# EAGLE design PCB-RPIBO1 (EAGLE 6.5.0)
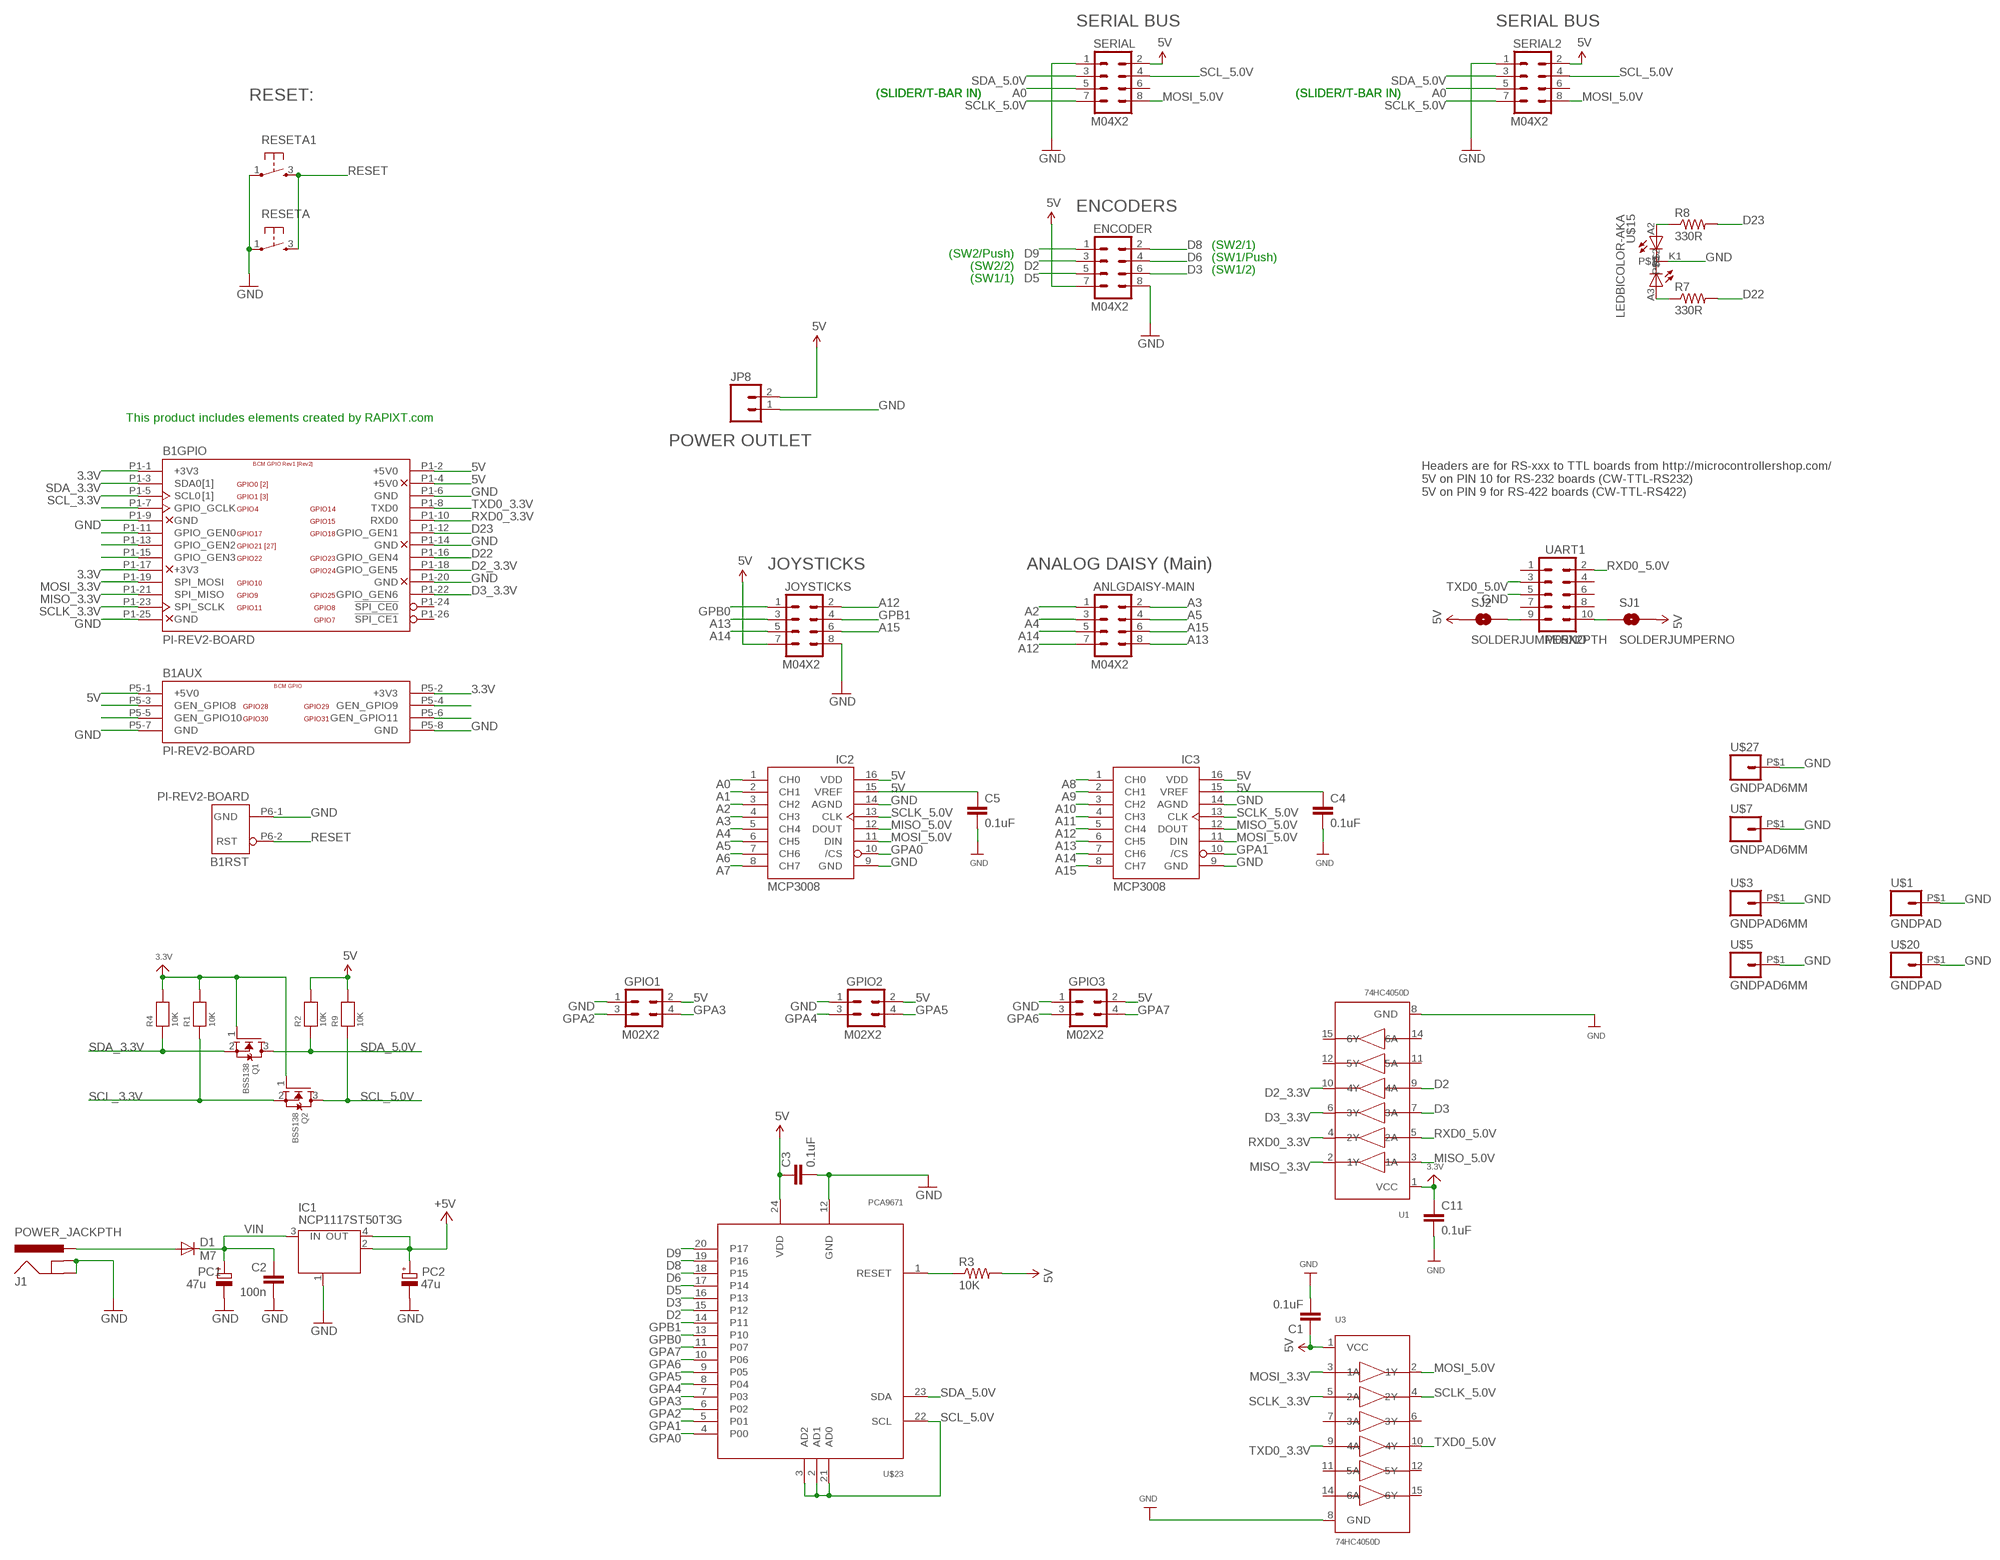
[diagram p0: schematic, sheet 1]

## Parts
ANLGDAISY-MAIN  M04X2  [2X4]
B1  PI-REV2-BOARD  [RASPBERRY-PI-REV2]
C1  0.1uF  CAP0603-CAP  [0603-CAP]
C2  100n  C-EU0603-RND  [C0603-ROUND]
C3  0.1uF  CAP0603-CAP  [0603-CAP]
C4  0.1uF  CAP0603-CAP  [0603-CAP]
C5  0.1uF  CAP0603-CAP  [0603-CAP]
C11  0.1uF  CAP0603-CAP  [0603-CAP]
D1  M7  DIODE-SMB  [SMB]
ENCODER  M04X2  [2X4]
GPIO1  M02X2  [2X2]
GPIO2  M02X2  [2X2]
GPIO3  M02X2  [2X2]
IC1  NCP1117ST50T3G  MC33269ST-3.3T3  [SOT223]
IC2  MCP3008  [DIL16]
IC3  MCP3008  [DIL16]
J1  POWER_JACKPTH  [POWER_JACK_PTH]
JOYSTICKS  M04X2  [2X4]
JP8  M02PTH4  [1X02_XTRA_BIG]
PC1  47u  CPOL-EUD  [PANASONIC_D]
PC2  47u  CPOL-EUD  [PANASONIC_D]
Q1  BSS138  MOSFET-NWIDE  [SOT23-WIDE]
Q2  BSS138  MOSFET-NWIDE  [SOT23-WIDE]
R1  10K  RESISTOR0805  [0805]
R2  10K  RESISTOR0805  [0805]
R3  10K  RESISTOR0603-RES  [0603-RES]
R4  10K  RESISTOR0805  [0805]
R7  330R  RESISTOR0603-RES  [0603-RES]
R8  330R  RESISTOR0603-RES  [0603-RES]
R9  10K  RESISTOR0805  [0805]
RESETA  TAC_SWITCH  [PUSHBUTTON]
RESETA1  TAC_SWITCH  [PUSHBUTTON]
SERIAL  M04X2  [2X4]
SERIAL2  M04X2  [2X4]
SJ1  SOLDERJUMPERNO  [SJ_2S-NO]
SJ2  SOLDERJUMPERNO  [SJ_2S-NO]
U1  74HC4050D  [SOIC16]
U3  74HC4050D  [SOIC16]
U$1  GNDPAD  [3.2MMPAD]
U$3  GNDPAD6MM  [3.2MMPAD6MM]
U$5  GNDPAD6MM  [3.2MMPAD6MM]
U$7  GNDPAD6MM  [3.2MMPAD6MM]
U$15  LEDBICOLOR-AKA  [LED5MM-BICOLOR]
U$20  GNDPAD  [3.2MMPAD]
U$23  PCA9671  [TSSOP24]
U$27  GNDPAD6MM  [3.2MMPAD6MM]
UART1  M05X2PTH  [AVR_ICSP]

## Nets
3.3V [Power]: B1.P1-1(GPIO:+3V3) B1.P1-17(GPIO:+3V3) B1.P5-2(AUX:+3V3) C11.1 Q1.1(G) Q2.1(G) R1.2 R4.2 U1.1(VCC)
5V [Power]: B1.P1-2(GPIO:+5V0) B1.P1-4(GPIO:+5V0) B1.P5-1(AUX:+5V0) C1.1 C3.1 C4.1 C5.1 ENCODER.7 GPIO1.2 GPIO2.2 GPIO3.2 IC1.2(OUT) IC1.4(OUT) IC2.15(VREF) IC2.16(VDD) IC3.15(VREF) IC3.16(VDD) JOYSTICKS.7 JP8.2 PC2.+ R2.2 R3.2 R9.2 SERIAL2.2 SERIAL.2 SJ1.2 SJ2.1 U3.1(VCC) U$23.24(VDD) ; supply symbol labelled +5V
12V [Power]: D1.A J1.PWR
A0: IC2.1(CH0) SERIAL2.5 SERIAL.5
A1: IC2.2(CH1)
A2: ANLGDAISY-MAIN.1 IC2.3(CH2)
A3: ANLGDAISY-MAIN.2 IC2.4(CH3)
A4: ANLGDAISY-MAIN.3 IC2.5(CH4)
A5: ANLGDAISY-MAIN.4 IC2.6(CH5)
A6: IC2.7(CH6)
A7: IC2.8(CH7)
A8: IC3.1(CH0)
A9: IC3.2(CH1)
A10: IC3.3(CH2)
A11: IC3.4(CH3)
A12: ANLGDAISY-MAIN.7 IC3.5(CH4) JOYSTICKS.2
A13: ANLGDAISY-MAIN.8 IC3.6(CH5) JOYSTICKS.3
A14: ANLGDAISY-MAIN.5 IC3.7(CH6) JOYSTICKS.5
A15: ANLGDAISY-MAIN.6 IC3.8(CH7) JOYSTICKS.6
D2: ENCODER.3 U1.9(4A) U$23.15(P12)
D2_3.3V: B1.P1-18(GPIO:GPIO_GEN5) U1.10(4Y)
D3: ENCODER.6 U1.7(3A) U$23.16(P13)
D3_3.3V: B1.P1-22(GPIO:GPIO_GEN6) U1.6(3Y)
D5: ENCODER.5 U$23.17(P14)
D6: ENCODER.4 U$23.18(P15)
D8: ENCODER.2 U$23.19(P16)
D9: ENCODER.1 U$23.20(P17)
D22: B1.P1-16(GPIO:GPIO_GEN4) R7.2
D23: B1.P1-12(GPIO:GPIO_GEN1) R8.2
GND [Power]: B1.P1-6(GPIO:GND) B1.P1-9(GPIO:GND) B1.P1-14(GPIO:GND) B1.P1-20(GPIO:GND) B1.P1-25(GPIO:GND) B1.P5-7(AUX:GND) B1.P5-8(AUX:GND) B1.P6-1(RST:GND) C1.2 C2.2 C3.2 C4.2 C5.2 C11.2 ENCODER.8 GPIO1.1 GPIO2.1 GPIO3.1 IC1.1(GND/ADJ) IC2.9(GND) IC2.14(AGND) IC3.9(GND) IC3.14(AGND) J1.GND J1.SHUNT(GNDBREAK) JOYSTICKS.8 JP8.1 PC1.- PC2.- RESETA1.1 RESETA.1 SERIAL2.1 SERIAL.1 U1.8(GND) U3.8(GND) U$1.P$1 U$3.P$1 U$5.P$1 U$7.P$1 U$15.K1 U$20.P$1 U$23.12(GND) U$27.P$1 UART1.5
GPA0: IC2.10(/CS) U$23.4(P00)
GPA1: IC3.10(/CS) U$23.5(P01)
GPA2: GPIO1.3 U$23.6(P02)
GPA3: GPIO1.4 U$23.7(P03)
GPA4: GPIO2.3 U$23.8(P04)
GPA5: GPIO2.4 U$23.9(P05)
GPA6: GPIO3.3 U$23.10(P06)
GPA7: GPIO3.4 U$23.11(P07)
GPB0: JOYSTICKS.1 U$23.13(P10)
GPB1: JOYSTICKS.4 U$23.14(P11)
MISO_3.3V: B1.P1-21(GPIO:SPI_MISO) U1.2(1Y)
MISO_5.0V: IC2.12(DOUT) IC3.12(DOUT) U1.3(1A)
MOSI_3.3V: B1.P1-19(GPIO:SPI_MOSI) U3.3(1A)
MOSI_5.0V: IC2.11(DIN) IC3.11(DIN) SERIAL2.8 SERIAL.8 U3.2(1Y)
N$1: R3.1 U$23.1(RESET)
N$9: SJ2.2 UART1.9
N$10: SJ1.1 UART1.10
N$17: R8.1 U$15.A2
N$22: R7.1 U$15.A3
N$23: B1.P1-15(GPIO:GPIO_GEN3)
N$24: B1.P1-13(GPIO:GPIO_GEN2)
N$25: B1.P1-11(GPIO:GPIO_GEN0)
N$27: B1.P1-7(GPIO:GPIO_GCLK)
N$34: B1.P5-4(AUX:GEN_GPIO9)
N$35: B1.P5-6(AUX:GEN_GPIO11)
N$38: B1.P5-3(AUX:GEN_GPIO8)
N$39: B1.P5-5(AUX:GEN_GPIO10)
RESET: B1.P6-2(RST:RST) RESETA1.3 RESETA.3
RXD0_3.3V: B1.P1-10(GPIO:RXD0) U1.4(2Y)
RXD0_5.0V: U1.5(2A) UART1.2
SCL_3.3V: B1.P1-5(GPIO:SCL0) Q2.2(S) R1.1
SCL_5.0V: Q2.3(D) R9.1 SERIAL2.4 SERIAL.4 U$23.2(AD1) U$23.3(AD2) U$23.21(AD0) U$23.22(SCL)
SCLK_3.3V: B1.P1-23(GPIO:SPI_SCLK) U3.5(2A)
SCLK_5.0V: IC2.13(CLK) IC3.13(CLK) SERIAL2.7 SERIAL.7 U3.4(2Y)
SDA_3.3V: B1.P1-3(GPIO:SDA0) Q1.2(S) R4.1
SDA_5.0V: Q1.3(D) R2.1 SERIAL2.3 SERIAL.3 U$23.23(SDA)
TXD0_3.3V: B1.P1-8(GPIO:TXD0) U3.9(4A)
TXD0_5.0V: U3.10(4Y) UART1.3
VIN [Power]: C2.1 D1.C IC1.3(IN) PC1.+
Unconnected: B1.P1-24(GPIO:!SPI_CE0) B1.P1-26(GPIO:!SPI_CE1) SERIAL2.6 SERIAL.6 U1.11(5A) U1.12(5Y) U1.14(6A) U1.15(6Y) U3.6(3Y) U3.7(3A) U3.11(5A) U3.12(5Y) U3.14(6A) U3.15(6Y) UART1.1 UART1.4 UART1.6 UART1.7 UART1.8

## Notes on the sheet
- SERIAL BUS | SERIAL BUS
- (SLIDER/T-BAR IN) | (SLIDER/T-BAR IN) | (SLIDER/T-BAR IN) | (SLIDER/T-BAR IN)
- RESET:
- ENCODERS
- (SW2/Push) | (SW2/1)
- (SW2/2) | (SW1/Push)
- (SW1/1) | (SW1/2)
- This product includes elements created by RAPIXT.com
- POWER OUTLET
- Headers are for RS-xxx to TTL boards from http://microcontrollershop.com/
  5V on PIN 10 for RS-232 boards (CW-TTL-RS232)
  5V on PIN 9 for RS-422 boards (CW-TTL-RS422)
- JOYSTICKS | ANALOG DAISY (Main)

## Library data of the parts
ANLGDAISY-MAIN ENCODER JOYSTICKS SERIAL SERIAL2 = SparkFun:M04X2
B1 = SKAARHOJ:PI-REV2-: Raspberry Pi Rev2
C1 C3-C5 C11 = SparkFun:CAP: Capacitor
C2 = SmartPrj:C-EU: CAPACITOR, European symbol
D1 = diode:DIODE-: DIODE
GPIO1-GPIO3 = SKAARHOJ:M02X2
IC1 = linear:MC33269ST*: Adjustable Output Low Dropout Voltage Regulator 800 mA Source: http://www.onsemi.com/pub/Collateral/MC33269-D.PDF
IC2 IC3 = adafruit:MCP3008
J1 = SKAARHOJ:POWER_JACK: RASM712PX Right Angle SMT Mount DC Power Jack, pin size 0.100"(2.5mm), with locating post Switchcraft.com
JP8 = SparkFun:M02: Header 2
PC1 PC2 = rcl:CPOL-EU: POLARIZED CAPACITOR, European symbol
Q1 Q2 = microbuilder:MOSFET-N: N-Channel Mosfet LEGEND VDS: Voltage Drain-Source ID: Drain Current RDS(ON): Drain-Source On-State Resistance VGS(TH): Gate-Source Threshold Voltage CISS: Drain-Source Input Capacitance SOT-23 Name VDS ID RDS(ON) VGS(TH) CISS Order Number 2N7002E 60V 260mA 2.5 Ohm 2.5V @ 250uA 26.7pF @ 25V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
R1 R2 R4 R9 = microbuilder:RESISTOR: Resistors
R3 R7 R8 = SparkFun:RESISTOR: Resistor
RESETA RESETA1 = SKAARHOJ:TAC_SWITCH: Momentary Switch
SJ1 SJ2 = SparkFun:SOLDERJUMPER: Solder Jumper
U1 U3 = microbuilder:74HC4050D: 6-channel level shifter 74HC4050D - 2V-6V Supply Digikey: 74HC4050D,653-ND Mouser: 771-74HC4050D-T
U$1 U$3 U$5 U$7 U$20 U$27 = SKAARHOJ:GNDPAD
U$15 = SKAARHOJ:LEDBICOLOR-AKA
U$23 = SKAARHOJ:PCA9671
UART1 = SparkFun:M05X2: Header 5x2 Standard 10-pin dual row 0.1" header. Commonly used with AVR-ISP. Use with Spark Fun Electronics SKU: PRT-00778

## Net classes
0 default: width 0.203 mm, drill 0.406 mm, clearance 0.152 mm
1 Power: width 0.508 mm, drill 0.61 mm, clearance 0.203 mm
3 INput lines: clearance 0.203 mm

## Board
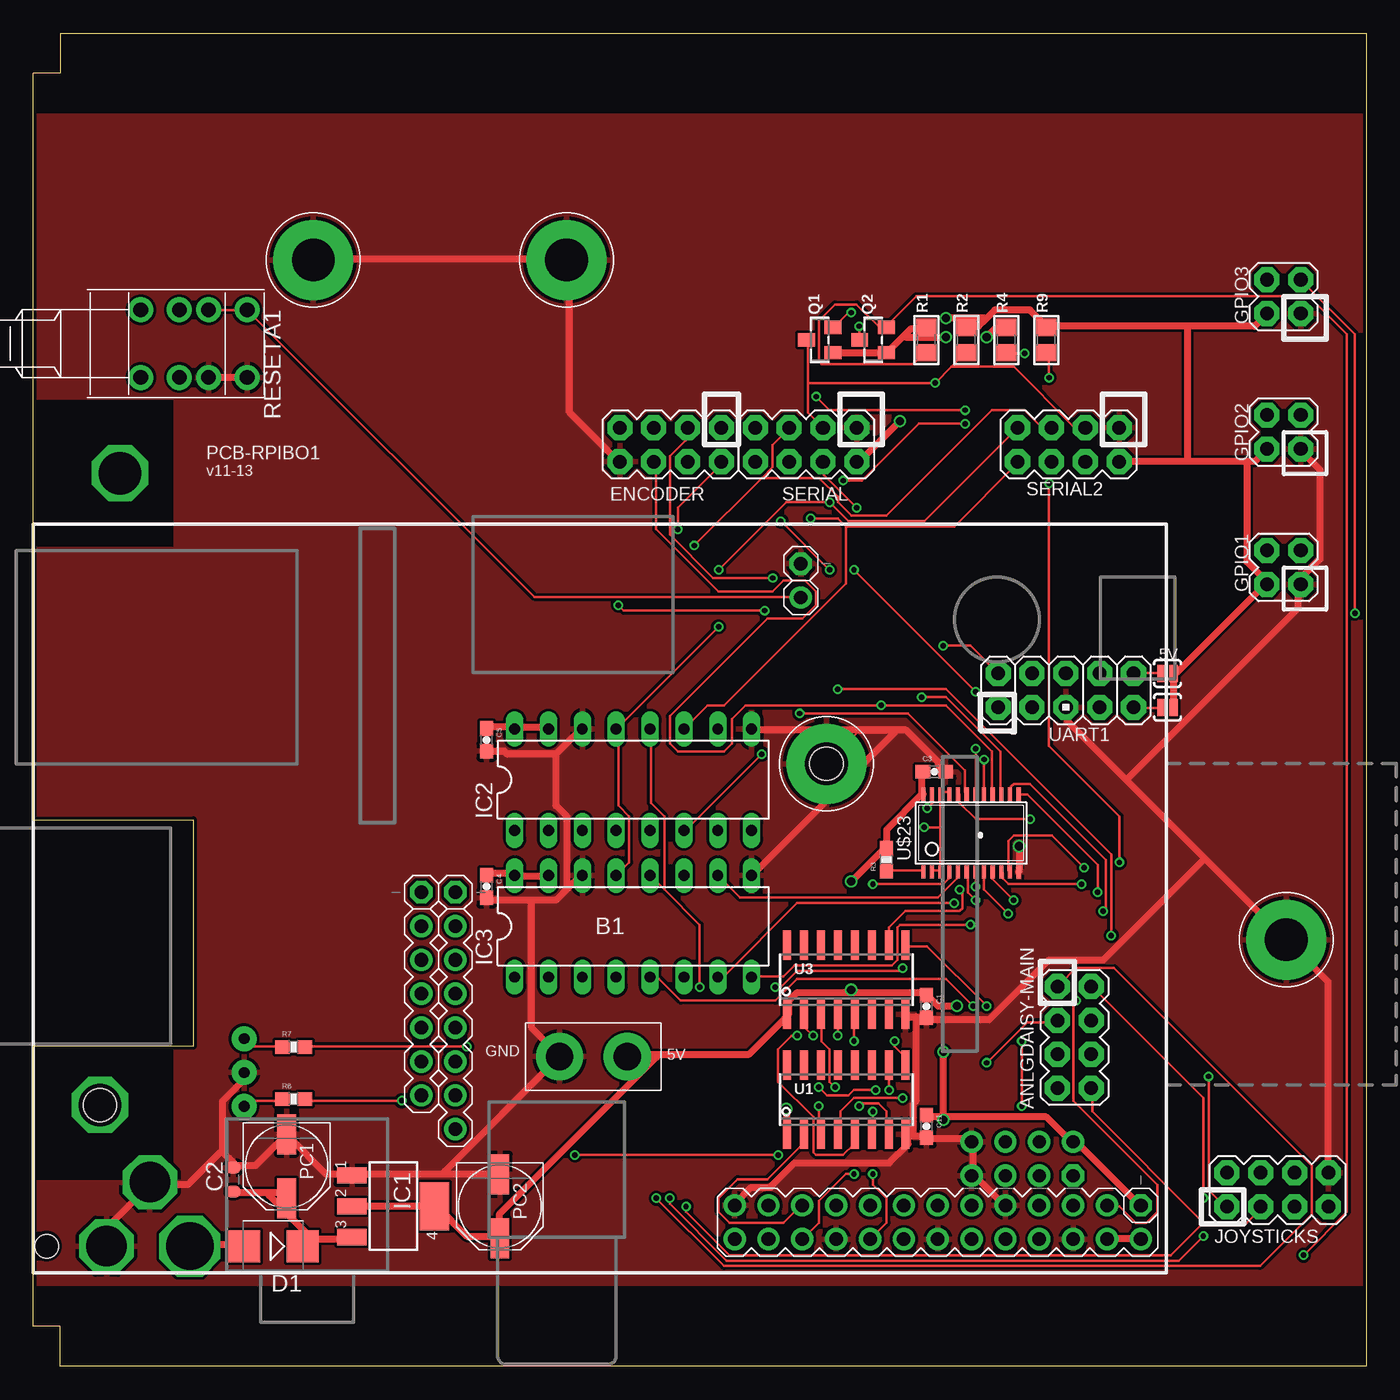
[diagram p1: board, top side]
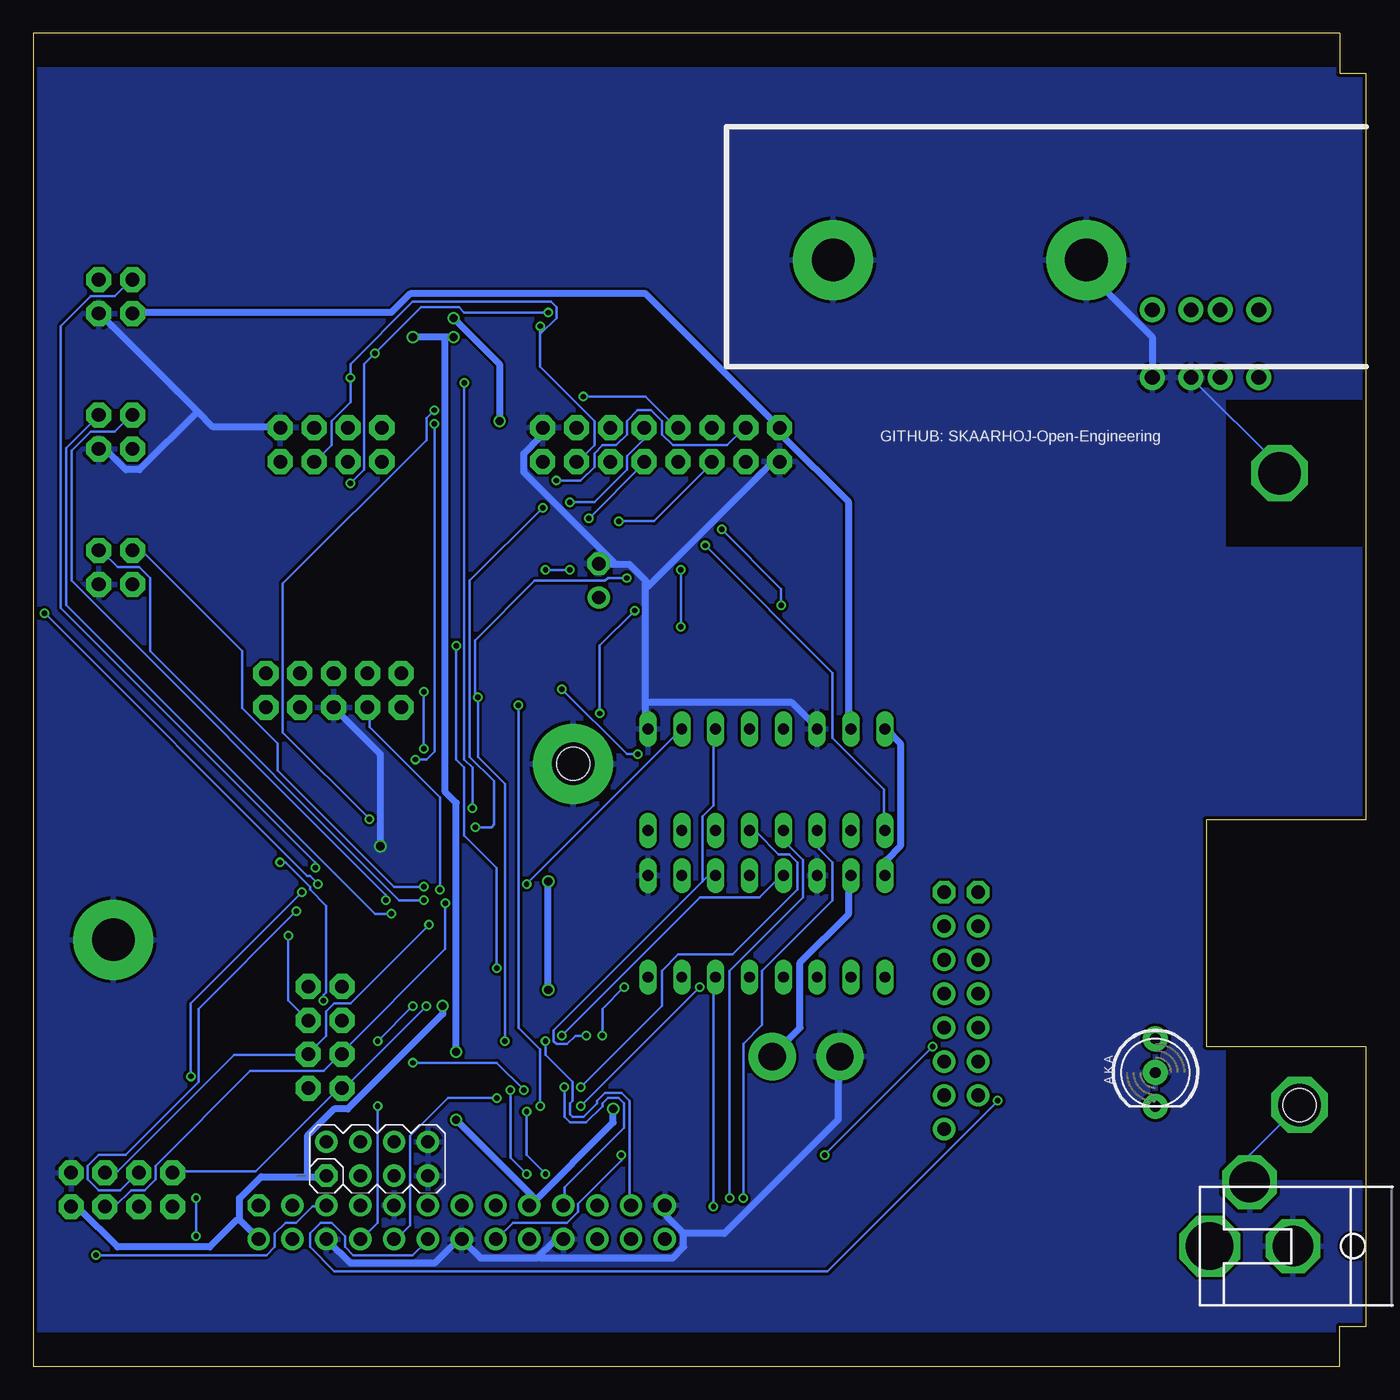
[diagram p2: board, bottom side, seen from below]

Size 100 x 100 mm. Coordinates in mm from the lower left corner, seen from the top.
Outline: 0,3 0,24 12,24 12,41 0,41 0,97 2,97 2,100 100,100 100,0 2,0 2,3 0,3
Copper layers (1*16): Top 0.035mm / dielectric 1.5mm / Bottom 0.035mm
Design rules "Fusion_eagle_rule_v1.1": minimum track width 6mil, minimum drill 12mil, track to track 6mil, track to pad 6mil, pad to pad 6mil, via to via 6mil, smd to smd 0mil, copper to edge 10mil, drill to drill 10mil, minimum pad ring 10mil, minimum via ring 6mil, stop-mask expansion 2mil, vias tented up to drill 100mil, thermal gap 10mil
tRestrict: area 0,14 to 10.5,25; area 0,61.5 to 10.5,72.5; area 0,94 to 100,100; area 0,0 to 100,6
bRestrict: area 0,61.5 to 10.5,72.5; area 0,14 to 10.5,25; area 0,0 to 100,2.5; area 0,97.5 to 100,100

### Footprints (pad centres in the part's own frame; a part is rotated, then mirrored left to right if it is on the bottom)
2X4 = drill 1.016 pad 1.88 octagon: 1 -3.81,-1.27; 2 -3.81,1.27; 3 -1.27,-1.27; 4 -1.27,1.27; 5 1.27,-1.27; 6 1.27,1.27; 7 3.81,-1.27; 8 3.81,1.27
RASPBERRY-PI-REV2 = drill 1.016 pad 1.676 octagon: P1-1 83.095,5.065; P2-1 31.66,28.56; P3-1 29.12,28.56 | drill 1.016 pad 1.676: P1-2 83.095,2.525; P1-3 80.555,5.065; P1-4 80.555,2.525; P1-5 78.015,5.065; P1-6 78.015,2.525; P1-7 75.475,5.065; P1-8 75.475,2.525; P1-9 72.935,5.065; P1-10 72.935,2.525; P1-11 70.395,5.065; P1-12 70.395,2.525; P1-13 67.855,5.065; P1-14 67.855,2.525; P1-15 65.315,5.065; P1-16 65.315,2.525; P1-17 62.775,5.065; P1-18 62.775,2.525; P1-19 60.235,5.065; P1-20 60.235,2.525; P1-21 57.695,5.065; P1-22 57.695,2.525; P1-23 55.155,5.065; P1-24 55.155,2.525; P1-25 52.615,5.065; P1-26 52.615,2.525; P2-2 31.66,26.02; P2-3 31.66,23.48; P2-4 31.66,20.94; P2-5 31.66,18.4; P2-6 31.66,15.86; P2-7 31.66,13.32; P2-8 31.66,10.78; P3-2 29.12,26.02; P3-3 29.12,23.48; P3-4 29.12,20.94; P3-5 29.12,18.4; P3-6 29.12,15.86; P3-7 29.12,13.32 | drill 1 pad 1.676 octagon: P5-1 78.015,7.287; P6-1 57.58,53.21 | drill 1 pad 1.676: P5-2 78.015,9.828; P5-3 75.475,7.287; P5-4 75.475,9.828; P5-5 72.935,7.287; P5-6 72.935,9.828; P5-7 70.395,7.287; P5-8 70.395,9.828; P6-2 57.58,50.67 | hole 2.5: 59.5,38.2; 5,12.6
0603-CAP = smd 1.1 x 1: 1 -0.85,0; 2 0.85,0
C0603-ROUND = smd 0.898 x 1.1: 1 -0.889,0; 2 0.889,0
SMB = smd 2.4 x 2.4: A 2.2,0; C -2.2,0
2X2 = drill 1.016 pad 1.88 octagon: 1 -3.81,-1.27; 2 -3.81,1.27; 3 -1.27,-1.27; 4 -1.27,1.27
SOT223 = smd 1.219 x 2.235: 1 -2.311,-3.099; 2 0,-3.099; 3 2.311,-3.099 | smd 3.6 x 2.2: 4 0,3.099
DIL16 = drill 0.813 long: 1 -8.89,-3.81; 2 -6.35,-3.81; 3 -3.81,-3.81; 4 -1.27,-3.81; 5 1.27,-3.81; 6 3.81,-3.81; 7 6.35,-3.81; 8 8.89,-3.81; 9 8.89,3.81; 10 6.35,3.81; 11 3.81,3.81; 12 1.27,3.81; 13 -1.27,3.81; 14 -3.81,3.81; 15 -6.35,3.81; 16 -8.89,3.81
POWER_JACK_PTH = drill 3.048 octagon: GND -7.493,0; SHUNT -10.744,4.801 | drill 3.556 octagon: PWR -13.741,0 | hole 1.778: -2.997,0
1X02_XTRA_BIG = drill 2.057 pad 3.556: 1 -2.54,0; 2 2.54,0
PANASONIC_D = smd 3 x 1.4: + 2.4,0; - -2.4,0
SOT23-WIDE = smd 1 x 1.27: 1 -0.95,-1; 2 0.95,-1; 3 0,1
0805 = smd 1.3 x 1.5: 1 -0.95,0; 2 0.95,0
0603-RES = smd 1.1 x 1: 1 -0.85,0; 2 0.85,0
PUSHBUTTON = drill 1.1 pad 1.88: 1 2.54,2.54; 2 2.54,-2.54; 3 -2.54,2.54; 4 -2.54,-2.54
SJ_2S-NO = smd 0.635 x 1.27: 1 -0.45,0; 2 0.45,0
SOIC16 = smd 0.6 x 2.2: 1 -4.445,-2.6; 2 -3.175,-2.6; 3 -1.905,-2.6; 4 -0.635,-2.6; 5 0.635,-2.6; 6 1.905,-2.6; 7 3.175,-2.6; 8 4.445,-2.6; 9 4.445,2.6; 10 3.175,2.6; 11 1.905,2.6; 12 0.635,2.6; 13 -0.635,2.6; 14 -1.905,2.6; 15 -3.175,2.6; 16 -4.445,2.6
3.2MMPAD = drill 3.2 octagon: P$1 0,0
3.2MMPAD6MM = drill 3.2 pad 6: P$1 0,0
LED5MM-BICOLOR = drill 0.813 pad 1.88: A2 2.54,0; A3 -2.54,0; K1 0,0
TSSOP24 = smd 0.305 x 0.991: 1 -4.225,-2.918; 2 -3.575,-2.918; 3 -2.925,-2.918; 4 -2.275,-2.918; 5 -1.625,-2.918; 6 -0.975,-2.918; 7 -0.325,-2.918; 8 0.325,-2.918; 9 0.975,-2.918; 10 1.625,-2.918; 11 2.275,-2.918; 12 2.925,-2.918; 13 2.925,2.918; 14 2.275,2.918; 15 1.625,2.918; 16 0.975,2.918; 17 0.325,2.918; 18 -0.325,2.918; 19 -0.975,2.918; 20 -1.625,2.918; 21 -2.275,2.918; 22 -2.925,2.918; 23 -3.575,2.918; 24 -4.225,2.918
AVR_ICSP = drill 1.016 pad 1.88 octagon: 1 -1.27,5.08; 2 1.27,5.08; 3 -1.27,2.54; 4 1.27,2.54; 5 -1.27,0; 6 1.27,0; 7 -1.27,-2.54; 8 1.27,-2.54; 9 -1.27,-5.08; 10 1.27,-5.08

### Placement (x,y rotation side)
ANLGDAISY-MAIN  78.11,24.67 270 top
B1  0,7 0 top
C1  67,27 270 top
C2  15,14 90 top
C3  67.6,44.6 0 top
C4  34,36 270 top
C5  34,47 270 top
C11  67,18 270 top
D1  18,9 180 top
ENCODER  47.81,69.14 180 top
GPIO1  93.83,62.47 90 top
GPIO2  93.83,72.63 90 top
GPIO3  93.83,82.79 90 top
IC1  27,12 270 top
IC2  45,44 0 top
IC3  45,33 0 top
J1  -2,9 0 bottom
JOYSTICKS  93.36,13.24 0 top
JP8  42.02,23.23 0 top
PC1  19,15 270 top
PC2  35,12 270 top
Q1  59,77 90 top
Q2  63,77 90 top
R1  67,77 90 top
R2  70,77 90 top
R3  64,38 90 top
R4  73,77 90 top
R7  19.52,23.95 0 top
R8  19.52,20.05 0 top
R9  76,77 90 top
RESETA  10.6,76.72 270 top
RESETA1  13.5,76.72 270 top
SERIAL  57.98,69.14 180 top
SERIAL2  77.66,69.14 180 top
SJ1  85.09,51.98 0 top
SJ2  85.09,49.44 180 top
U1  61,20 0 top
U3  61,29 0 top
U$1  6.5,67 0 top
U$3  21,83 0 top
U$5  40,83 0 top
U$7  94,32 0 top
U$15  15.81,22.03 270 bottom
U$20  5,19.6 0 top
U$23  71,40 0 top
U$27  59.5,45.2 0 top
UART1  77.47,50.7 90 top

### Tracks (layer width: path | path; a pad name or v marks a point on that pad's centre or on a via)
3.3V  (via drill 0.61)
  Top 0.508: v56.49,19.3 56.49,17.48 U1.1 | Q1.1 60.15,76 63.8,76 Q2.1 64.21,76.2 65.33,77.32 | 65.33,77.32 65.84,77.83 66.85,77.83 R1.2 | v71.53,77.22 72.14,77.83 72.95,77.83 R4.2 | v68.48,77.22 65.43,77.22 65.33,77.32 | 68.28,18.69 76,18.69 77.83,16.87 B1.P5-2 78.23,16.87 82.91,12.19 B1.P1-1 | 68.28,18.69 67.06,18.69 C11.1 | 68.28,18.69 v68.28,23.57 | v68.28,18.49 68.28,18.69
  Bottom 0.508: v56.49,19.3 56.49,18.29 62.59,12.19 B1.P1-17 62.38,12.6 v68.28,18.49 | v68.48,77.22 69.09,77.22 | 69.09,77.22 v71.53,77.22 | 69.09,77.22 69.09,43.08 68.28,42.27 v68.28,23.57
5V  (via drill 0.61)
  Top 0.508: SJ2.1 85.55,49.58 85.55,51.82 SJ1.2 85.75,52.02 92.46,58.73 GPIO1.2 92.46,58.93 91.03,60.35 91.03,67.87 | 91.03,67.87 91.64,67.87 92.46,68.68 GPIO2.2 | 91.03,67.87 86.56,67.87 | 86.56,67.87 81.48,67.87 SERIAL2.2 | 71.42,78.54 72.14,79.25 74.78,79.25 76,78.03 R9.2 76.2,78.03 86.56,78.03 | 71.42,78.54 70.92,78.03 70.1,78.03 R2.2 | 86.56,78.03 91.64,78.03 92.46,78.84 GPIO3.2 | v65.02,70.92 61.98,67.87 SERIAL.2 | v68.48,78.64 71.32,78.64 71.42,78.54 | 86.56,78.03 86.56,67.87 | C4.1 34.14,36.98 35.97,36.98 IC3.16 36.17,36.78 38.61,36.78 IC3.15 | C5.1 34.14,47.95 35.97,47.95 IC2.16 36.17,47.95 38.61,47.95 IC2.15 | B1.P1-4 80.67,9.55 82.91,9.55 B1.P1-2 | IC1.2 23.98,11.99 30.07,11.99 IC1.4 30.28,11.99 32.51,9.75 34.95,9.75 PC2.+ 34.95,9.96 34.95,11.38 46.74,23.16 46.74,23.37 | C3.1 66.65,44.5 66.65,43.08 U$23.24 66.65,42.88 64.01,40.23 64.01,39.01 R3.2 63.8,38.81 v61.37,36.37 | 61.37,28.04 57.3,28.04 56.69,27.43 56.69,26.42 U3.1 56.49,26.21 53.65,23.37 46.74,23.37 | 61.37,28.04 66.85,28.04 C1.1 67.06,27.84 67.87,27.03 v69.29,27.03 | v61.37,28.25 61.37,28.04 | 46.74,23.37 44.7,23.37 JP8.2
  Bottom 0.508: v65.02,70.92 65.02,75.18 v68.48,78.64 | IC2.15 38.81,47.95 38.81,64.82 43.89,69.9 43.89,70.31 ENCODER.7 44.09,70.51 54.05,80.47 71.73,80.47 73.15,79.05 92.46,79.05 GPIO3.2 | IC3.16 35.97,36.98 35.97,38 34.95,39.01 34.95,46.74 35.97,47.75 IC2.16 | 79.45,14.22 82.91,14.22 84.53,12.6 84.53,10.97 | 79.45,14.22 78.03,14.22 B1.P5-1 | 84.53,10.97 83.11,9.55 B1.P1-2 | JOYSTICKS.7 97.13,11.79 96.52,11.79 93.67,8.94 86.77,8.94 84.73,10.97 84.53,10.97 | v61.37,28.25 v61.37,36.37 | 79.45,14.22 79.45,17.27 77.42,19.3 76.4,19.3 69.29,26.42 v69.29,27.03 | IC3.15 38.81,36.78 38.81,33.93 42.47,30.28 42.47,25.4 44.5,23.37 JP8.2
12V
  Top 0.508: D1.A 15.65,9.14 11.79,9.14 J1.PWR
A0  (via drill 0.41)
  Top 0.203: 54.66,66.65 55.47,67.46 55.47,69.09 56.69,70.31 SERIAL.5 | 54.66,66.65 v49.58,61.57 | 54.66,66.65 58.93,66.65 60.35,65.23 60.35,64.82 61.37,63.8 64.01,63.8 71.93,71.73 74.37,71.73 75.59,70.51 76.2,70.51 SERIAL2.5
  Bottom 0.203: v49.58,61.57 40.03,52.02 40.03,47.14 36.17,43.28 36.17,40.23 IC2.1
A2  (via drill 0.41)
  Top 0.203: v46.74,12.6 51.82,7.52 92.05,7.52 95.91,11.38 95.91,15.04 81.08,29.87 78.23,29.87 77.01,28.65 ANLGDAISY-MAIN.1
  Bottom 0.203: v46.74,12.6 46.74,24.18 45.31,25.6 45.31,29.67 40.03,34.95 40.03,37.8 41.05,38.81 41.05,40.03 IC2.3
A3  (via drill 0.41)
  Top 0.203: v47.75,12.6 47.75,12.19 52.02,7.92 85.95,7.92 v87.78,9.75 | v87.78,12.6 87.78,20.12 79.45,28.45 ANLGDAISY-MAIN.2
  Bottom 0.203: v47.75,12.6 47.75,29.67 42.27,35.15 42.27,38 43.69,39.42 43.69,40.03 IC2.4 | v87.78,12.6 v87.78,9.75
A4  (via drill 0.41)
  Top 0.203: v58.93,20.93 59.54,20.32 61.16,20.32 61.57,20.73 v63.2,20.73 | v71.53,22.76 74.57,25.81 76.81,25.81 ANLGDAISY-MAIN.3
  Bottom 0.203: v58.93,20.93 52.83,27.03 52.83,29.67 51.61,30.89 47.55,30.89 42.67,35.76 42.67,37.8 43.28,38.41 44.09,38.41 45.72,40.03 46.13,40.03 IC2.5 | v63.2,20.73 65.23,22.76 v71.53,22.76
A5  (via drill 0.41)
  Top 0.203: v54.66,45.92 48.97,40.23 IC2.6 | v60.35,50.8 68.48,50.8 80.87,38.41 v80.87,32.31
  Bottom 0.203: v54.66,45.92 55.47,45.92 v60.35,50.8 | v80.87,32.31 80.87,27.43 79.45,26.01 ANLGDAISY-MAIN.4
A12  (via drill 0.41)
  Top 0.203: v70.51,27.03 68.48,29.06 57.3,29.06 55.68,27.43 48.56,27.43 46.94,29.06 46.33,29.06 IC3.5
  Bottom 0.203: v70.51,27.03 76.81,20.73 ANLGDAISY-MAIN.7 77.01,20.93 83.31,14.63 89.41,14.63 JOYSTICKS.2
A13  (via drill 0.41)
  Top 0.203: v48.97,11.99 48.97,11.58 52.22,8.33 85.34,8.33 87.78,10.77 | 87.78,10.77 91.03,10.77 92.05,11.79 JOYSTICKS.3 | 87.78,10.77 79.45,19.1 79.45,20.73 ANLGDAISY-MAIN.8
  Bottom 0.203: v48.97,11.99 48.97,29.06 IC3.6
A14  (via drill 0.41)
  Top 0.203: v69.09,34.75 57.3,34.75 51.82,29.26 51.41,29.26 IC3.7
  Bottom 0.203: v69.09,34.75 69.09,31.29 76.81,23.57 ANLGDAISY-MAIN.5 77.01,23.37 78.23,22.15 83.72,22.15 90.83,15.04 90.83,14.02 91.64,13.21 92.66,13.21 93.88,11.99 94.49,11.99 JOYSTICKS.5
A15  (via drill 0.41)
  Top 0.203: v70.31,33.12 65.02,33.12 64.82,32.92 64.82,30.48 64.41,30.07 57.1,30.07 56.29,29.26 54.05,29.26 IC3.8
  Bottom 0.203: v70.31,33.12 76.2,27.23 77.42,27.23 78.03,26.62 78.03,24.79 79.25,23.57 ANLGDAISY-MAIN.6 79.45,23.37 84.94,23.37 93.67,14.63 94.49,14.63 JOYSTICKS.6
D2  (via drill 0.41)
  Top 0.203: v66.65,50.19 68.48,50.19 72.54,46.13 72.54,43.08 U$23.15 | v64.62,24.38 64.62,23.98 65.43,23.16 65.43,22.76 U1.9 | v55.47,59.13 51,59.13 47.75,62.38 47.75,68.28 48.97,69.49 48.97,70.31 ENCODER.3
  Bottom 0.203: v64.62,24.38 64.62,43.69 66.65,45.72 v66.65,50.19 66.85,50.39 66.85,54.46 62.38,58.93 57.1,58.93 56.9,59.13 v55.47,59.13
D2_3.3V  (via drill 0.41)
  Top 0.203: v64.21,20.73 64.21,22.55 U1.10 | v62.99,14.43 62.99,13.61 64.01,12.6 64.01,10.77 62.79,9.55 B1.P1-18
  Bottom 0.203: v64.21,20.73 64.21,15.65 v62.99,14.43
D3  (via drill 0.41)
  Top 0.203: U$23.16 71.93,43.08 71.93,46.13 68.48,49.58 v63.6,49.58 53.44,49.58 52.43,48.56 52.43,46.74 51.82,46.13 48.36,46.13 47.75,46.74 47.75,48.77 55.07,56.08 57.71,56.08 58.73,57.1 58.73,58.12 57.91,58.93 56.29,58.93 55.47,58.12 51.41,58.12 46.74,62.79 46.74,67.67 ENCODER.6 | v61.98,19.51 62.18,19.71 63.4,19.71 64.01,19.1 64.01,17.48 U1.7
  Bottom 0.203: v61.98,19.51 61.98,23.77 63.6,25.4 v63.6,49.58
D3_3.3V  (via drill 0.41)
  Top 0.203: v62.99,19.1 62.99,17.48 U1.6 | v61.57,14.43 60.96,14.43 58.93,12.39 58.93,10.77 57.71,9.55 B1.P1-22
  Bottom 0.203: v62.99,19.1 62.99,15.85 v61.57,14.43
D5  (via drill 0.41)
  Top 0.203: v71.32,45.52 71.32,43.08 U$23.17 | v69.9,70.71 66.45,70.71 62.18,66.45 v60.76,66.45
  Bottom 0.203: v71.32,45.52 70.51,45.52 69.9,46.13 v69.9,70.71 | v60.76,66.45 58.93,66.45 57.91,67.46 57.91,68.48 57.3,69.09 56.29,69.09 55.47,69.9 55.47,70.92 54.66,71.73 53.65,71.73 52.83,70.92 52.83,69.9 52.02,69.09 47.95,69.09 46.74,70.31 ENCODER.5
D6  (via drill 0.41)
  Top 0.203: v70.71,46.33 70.71,43.08 U$23.18 | v61.57,59.74 v70.71,50.6 | v56.08,63.4 v59.74,59.74
  Bottom 0.203: v70.71,50.6 v70.71,46.33 | v59.74,59.74 v61.57,59.74 | v56.08,63.4 53.44,63.4 49.17,67.67 ENCODER.4
D8  (via drill 0.41)
  Top 0.203: v57.51,48.97 65.63,48.97 69.9,44.7 69.9,43.08 U$23.19 | v54.86,56.69 44.3,56.69 v43.89,57.1 | v48.36,62.79 48.36,64.41 51.61,67.67 ENCODER.2
  Bottom 0.203: v57.51,48.97 57.51,54.05 v54.86,56.69 | v43.89,57.1 43.89,58.32 v48.36,62.79
D9  (via drill 0.41)
  Top 0.203: v74.78,41.05 70.71,41.05 69.49,42.27 69.49,42.88 U$23.20 | v69.9,71.73 59.74,71.73 v58.73,72.75
  Bottom 0.203: v74.78,41.05 81.28,47.55 81.28,58.73 70.51,69.49 70.51,71.12 v69.9,71.73 | v58.73,72.75 54.05,72.75 51.82,70.51 ENCODER.1
D22  (via drill 0.41)
  Top 0.203: v32.51,23.98 20.52,23.98 R7.2 | v55.88,15.85 v40.64,15.85
  Bottom 0.203: v40.64,15.85 v32.51,23.98 | v55.88,15.85 55.88,15.44 59.13,12.19 59.13,11.58 59.94,10.77 64.01,10.77 65.23,9.55 B1.P1-16
D23  (via drill 0.41)
  Top 0.203: v27.64,19.91 20.52,19.91 R8.2
  Bottom 0.203: v27.64,19.91 40.44,7.11 77.42,7.11 79.25,8.94 79.25,9.96 78.44,10.77 77.62,10.77 76.61,9.75 76.61,8.94 76,8.33 71.53,8.33 70.51,9.35 B1.P1-12
GND  (via drill 0.61)
  Top 0.203: 64.62,47.55 61.85,47.55 U$27.P$1
  Top 0.508: RESETA.1 13.21,74.17 15.85,74.17 RESETA1.1 | U$3.P$1 21.13,83.11 39.83,83.11 U$5.P$1 40.23,82.91 40.23,71.53 43.89,67.87 ENCODER.8 | 53.85,36.78 IC3.9 54.05,36.98 64.62,47.55 64.62,47.75 | 64.62,47.75 54.05,47.75 IC2.9 | 64.62,47.75 65.43,47.75 67.87,45.31 67.87,45.11 68.28,44.7 C3.2 | GPIO2.1 95.1,68.68 96.52,67.26 96.52,60.55 95.1,59.13 95.1,58.73 GPIO1.1 94.89,58.52 94.89,56.9 81.99,43.99 | 73.97,37.19 U$23.12 73.97,37.39 v73.97,39.01 | JOYSTICKS.8 97.13,14.63 97.13,28.85 94.08,31.9 U$7.P$1 93.88,32.11 87.88,38.1 | 87.88,38.1 81.99,43.99 | 81.99,43.99 77.62,48.36 77.62,49.38 UART1.5 | 66.24,26.21 65.63,26.21 U3.8 | 66.24,26.21 66.85,26.21 C1.2 67.06,26.01 71.73,26.01 76.2,30.48 80.26,30.48 87.88,38.1 | 66.04,17.27 65.63,17.27 U1.8 65.63,17.07 65.63,16.66 64.21,15.24 57.1,15.24 55.27,13.41 53.85,13.41 52.63,12.19 B1.P1-25 | 66.04,17.27 66.85,17.27 C11.2 67.26,17.07 70.1,17.07 70.31,16.87 B1.P5-8 70.51,16.66 70.51,14.43 | 66.24,26.21 66.24,19.91 66.04,19.71 66.04,17.27 | 70.51,14.43 72.75,12.19 B1.P1-9 | 70.51,14.43 B1.P5-7 | 39.22,45.92 35.56,45.92 35.36,46.13 34.14,46.13 C5.2 | 39.22,45.92 41.05,47.75 IC2.14 | 37.39,34.95 39.22,34.95 40.13,35.87 | 37.39,34.95 34.14,34.95 C4.2 | 40.13,35.87 41.05,36.78 IC3.14 | 37.39,34.95 37.39,25.4 39.42,23.37 JP8.1 39.42,23.16 30.89,14.63 30.89,14.43 | 39.22,45.92 39.22,42.06 40.03,41.25 40.03,35.97 40.13,35.87 | J1.GND 5.69,9.14 5.69,10.57 8.74,13.61 J1.SHUNT 8.94,13.61 11.58,13.61 14.02,16.05 14.22,16.05 | 30.89,14.43 23.98,14.43 IC1.1 23.77,14.43 21.95,14.43 19.1,17.27 PC1.- 18.9,17.27 16.66,15.04 15.04,15.04 C2.2 15.04,15.24 14.22,16.05
  Top 0.508: 30.89,14.43 34.95,14.43 PC2.- | 14.22,16.05 14.22,19.91 15.65,21.34 15.65,21.95 U$15.K1
  Bottom 0.203: J1.SHUNT 8.74,15.86 U$20.P$1 | U$1.P$1 6.5,67.54 RESETA.1
  Bottom 0.508: RESETA1.1 16.05,74.37 16.05,77.22 20.93,82.09 20.93,82.91 U$3.P$1 | 56.49,60.15 55.27,60.15 54.05,58.93 54.05,58.52 | 56.49,60.15 57.51,60.15 B1.P6-1 | 54.05,49.78 54.05,47.95 IC2.9 | 54.05,49.78 54.05,58.52 | ENCODER.8 44.09,67.67 44.7,67.67 53.85,58.52 54.05,58.52 | SERIAL.1 61.98,70.31 61.98,69.7 63.2,68.48 63.2,67.06 56.49,60.35 56.49,60.15 | 87.68,71.63 94.89,78.84 GPIO3.1 | 87.68,71.63 86.56,70.51 81.48,70.51 SERIAL2.1 | 87.68,71.63 92.05,67.26 93.07,67.26 94.49,68.68 94.89,68.68 GPIO2.1 | v73.97,39.01 73.97,45.92 77.42,49.38 UART1.5 | 62.08,8.23 62.18,8.13 66.45,8.13 67.67,9.35 B1.P1-14 68.07,9.55 69.9,7.72 76.2,7.72 77.83,9.35 B1.P1-6 | 62.08,8.23 60.96,9.35 60.35,9.35 B1.P1-20 | 51.21,9.96 52.43,11.18 52.43,11.99 B1.P1-25 | 51.21,9.96 51.21,8.94 52.02,8.13 61.98,8.13 62.08,8.23 | 51.21,9.96 48.16,9.96 39.62,18.49 39.62,23.16 JP8.1 | 54.05,49.78 43.08,49.78 41.25,47.95 IC2.14
  pour Top: 0,0 100,0 100,100 0,100
  pour Bottom: 0,0 100,0 100,100 0,100
GPA0  (via drill 0.41)
  Top 0.203: v62.99,36.17 68.28,36.17 68.68,36.58 68.68,36.98 U$23.4
  Bottom 0.203: v62.99,36.17 51.41,47.75 IC2.10
GPA1
  Top 0.203: U$23.5 69.29,36.98 69.29,36.58 67.87,35.15 53.03,35.15 51.41,36.78 IC3.10
GPA2  (via drill 0.41)
  Top 0.203: v70.71,34.95 70.1,35.56 70.1,36.98 U$23.6
  Bottom 0.203: v70.71,34.95 72.54,34.95 91.24,53.65 91.24,59.13 92.05,59.94 93.67,59.94 94.89,61.16 GPIO1.3
GPA3  (via drill 0.41)
  Top 0.203: v70.71,35.97 70.71,36.98 U$23.7
  Bottom 0.203: v70.71,35.97 72.95,35.97 81.69,44.7 81.69,46.74 84.33,49.38 84.33,53.65 91.85,61.16 92.46,61.16 GPIO1.4
GPA4  (via drill 0.41)
  Top 0.203: v73.15,33.93 71.32,35.76 71.32,36.98 U$23.8
  Bottom 0.203: v73.15,33.93 74.37,33.93 97.54,57.1 97.54,68.89 95.1,71.32 GPIO2.3
GPA5  (via drill 0.41)
  Top 0.203: v73.56,34.95 71.93,36.58 71.93,36.98 U$23.9
  Bottom 0.203: v73.56,34.95 73.56,35.36 97.13,58.93 97.13,68.68 95.71,70.1 93.88,70.1 92.66,71.32 GPIO2.4
GPA6  (via drill 0.41)
  Top 0.203: v78.64,36.17 73.15,36.17 72.75,36.58 72.75,36.98 U$23.10 | v99.16,56.49 99.16,77.42 95.1,81.48 GPIO3.3
  Bottom 0.203: v78.64,36.17 79.25,36.78 79.45,36.78 v99.16,56.49
GPA7  (via drill 0.41)
  Top 0.203: v78.84,37.39 76.4,39.83 73.56,39.83 73.15,39.42 73.15,37.19 U$23.11
  Bottom 0.203: v78.84,37.39 78.84,37.8 97.94,56.9 97.94,78.03 95.71,80.26 93.88,80.26 92.66,81.48 GPIO3.4
GPB0  (via drill 0.41)
  Top 0.203: v79.86,35.56 79.86,37.59 74.57,42.88 73.97,42.88 U$23.13 | v88.19,21.74 88.19,13.21 89.41,11.99 JOYSTICKS.1
  Bottom 0.203: v79.86,35.56 88.19,27.23 v88.19,21.74
GPB1  (via drill 0.41)
  Top 0.203: v80.26,34.14 80.47,34.34 80.47,38 74.78,43.69 73.56,43.69 73.36,43.48 73.36,43.08 U$23.14
  Bottom 0.203: v80.26,34.14 87.58,26.82 87.58,21.34 93.07,15.85 95.1,15.85 95.91,15.04 95.91,14.02 95.1,13.21 93.47,13.21 92.25,14.43 JOYSTICKS.4
MISO_3.3V
  Top 0.203: U1.2 57.71,17.27 57.71,16.66 55.07,14.02 52.83,14.02 51.41,12.6 51.41,11.58 52.22,10.77 56.29,10.77 57.51,11.99 B1.P1-21
MISO_5.0V  (via drill 0.41)
  Top 0.203: v58.93,19.51 58.93,17.48 U1.3 | v49.99,28.45 49.99,33.12 47.35,35.76 | 47.35,35.76 46.33,36.78 IC3.12 | 47.35,35.76 47.35,41.25 46.33,42.27 46.33,47.75 IC2.12
  Bottom 0.203: v49.99,28.45 v58.93,19.51
MOSI_3.3V  (via drill 0.41)
  Top 0.203: v60.15,20.93 59.74,21.34 59.74,23.77 59.13,24.38 59.13,26.21 U3.3
  Bottom 0.203: v60.15,20.93 60.15,18.69 59.74,18.29 58.52,18.29 57.3,19.51 57.3,19.71 56.9,20.12 56.08,20.12 55.68,19.71 55.68,17.88 60.15,13.41 60.15,12.19 B1.P1-19
MOSI_5.0V  (via drill 0.41)
  Top 0.203: v58.32,63.6 60.35,63.6 60.96,62.99 | 60.96,62.99 69.09,62.99 73.76,67.67 SERIAL2.8 | v58.52,24.79 57.91,25.4 57.91,26.21 U3.2 | 60.96,62.99 60.96,58.73 51.82,49.58 50.6,49.58 48.97,47.95 IC2.11
  Bottom 0.203: v58.32,63.6 54.25,67.67 SERIAL.8 | v58.52,24.79 59.33,24.79 59.94,24.18 60.76,24.18 60.96,24.38 60.96,25.2 49.78,36.37 | 49.78,36.37 49.38,36.78 48.97,36.78 IC3.11 | 49.78,36.37 49.78,41.25 48.97,42.06 48.97,47.75 IC2.11
N$1
  Top 0.203: U$23.1 66.65,37.19 64.01,37.19 R3.1
N$9
  Top 0.203: SJ2.2 84.53,49.38 82.7,49.38 UART1.9
N$10
  Top 0.203: SJ1.1 84.53,52.02 82.7,52.02 UART1.10
N$17
  Top 0.203: R8.1 18.49,19.91 16.26,19.91 15.85,19.51 U$15.A2
N$22
  Top 0.203: R7.1 18.49,23.98 16.26,23.98 15.85,24.38 U$15.A3
RESET
  Top 0.203: B1.P6-2 57.51,57.71 37.59,57.71 16.05,79.25 RESETA1.3 15.85,79.25 13.21,79.25 RESETA.3
RXD0_3.3V  (via drill 0.41)
  Top 0.203: v65.23,20.12 61.57,20.12 60.55,19.1 60.55,17.48 U1.4
  Bottom 0.203: v65.23,20.12 68.89,20.12 71.73,17.27 71.73,10.57 72.75,9.55 B1.P1-10
RXD0_5.0V  (via drill 0.41)
  Top 0.203: v57.3,24.79 56.9,24.79 55.88,23.77 55.88,21.34 58.52,18.69 58.52,16.05 58.73,15.85 60.76,15.85 61.57,16.66 61.57,17.27 U1.5 | v55.68,28.45 56.08,28.45 57.3,29.67 65.02,29.67 v65.23,29.87 | v68.28,54.05 70.31,54.05 72.34,52.02 UART1.2
  Bottom 0.203: v57.3,24.79 57.3,26.82 v55.68,28.45 | v65.23,29.87 65.23,37.39 67.67,39.83 67.67,44.91 68.28,45.52 v68.28,54.05
SCL_3.3V  (via drill 0.41)
  Top 0.203: R1.1 66.85,76 66.04,75.18 59.13,75.18 58.93,75.39 58.93,78.44 60.15,79.65 61.77,79.65 63.4,78.03 63.8,78.03 Q2.2 64.01,78.03 66.24,80.26 95.71,80.26 98.55,77.42 98.55,11.58 v95.3,8.33
  Bottom 0.203: v95.3,8.33 82.5,8.33 81.89,8.94 81.89,9.96 81.08,10.77 80.26,10.77 79.05,11.99 78.03,11.99 B1.P1-5
SCL_5.0V  (via drill 0.41)
  Top 0.203: v76.2,74.17 76.2,76 R9.1 | 68.07,37.19 67.46,37.19 U$23.2 | U$23.21 68.68,43.08 68.07,43.08 U$23.22 68.07,42.88 68.07,40.44 | 68.07,40.44 68.07,37.19 | 68.07,37.19 U$23.3 | v61.98,78.03 61.98,77.01 Q2.3 | v66.85,40.44 68.07,40.44 | v61.77,64.41 59.33,66.85 59.33,67.67 SERIAL.4
  Bottom 0.203: SERIAL2.4 78.84,67.87 77.62,69.09 77.62,70.92 76.2,72.34 v76.2,74.17 76.2,75.18 71.53,79.86 61.16,79.86 60.76,79.45 60.76,78.64 61.98,77.42 | 61.98,77.42 61.98,74.98 57.91,70.92 57.91,69.09 59.13,67.87 SERIAL.4 | 61.98,77.42 v61.98,78.03 | v66.85,40.44 65.63,40.44 65.43,40.64 65.43,43.89 67.26,45.72 67.26,58.93 v61.77,64.41
SCLK_3.3V  (via drill 0.41)
  Top 0.203: v61.57,24.38 61.57,26.21 U3.5
  Bottom 0.203: v61.57,24.38 61.57,23.37 59.54,21.34 59.54,19.91 59.74,19.71 59.74,18.9 59.54,18.69 58.73,18.69 57.71,19.71 57.71,19.91 57.1,20.52 55.88,20.52 55.27,19.91 55.27,12.19 B1.P1-23
SCLK_5.0V  (via drill 0.41)
  Top 0.203: SERIAL2.7 73.76,70.31 66.85,63.4 61.16,63.4 v59.74,64.82 56.49,64.82 v51.41,59.74 | v60.35,24.79 60.35,26.21 U3.4 | IC3.13 43.89,36.98 44.7,37.8 44.7,41.25 43.89,42.06 43.89,47.75 IC2.13 43.89,47.95 v51.41,55.47
  Bottom 0.203: v59.74,64.82 57.91,64.82 55.47,67.26 55.47,68.28 54.25,69.49 54.25,70.31 SERIAL.7 | v60.35,24.79 49.99,35.15 45.52,35.15 43.89,36.78 IC3.13 | v51.41,55.47 v51.41,59.74
SDA_3.3V  (via drill 0.41)
  Top 0.203: v61.37,79.05 61.16,79.05 60.15,78.03 Q1.2 | v74.37,76 73.15,76 R4.1 | v78.23,27.43 78.03,27.23 78.03,19.91 84.33,13.61 84.33,11.58 83.52,10.77 82.7,10.77 81.48,11.99 80.67,11.99 B1.P1-3 | v81.48,37.8 81.48,41.25 76.2,46.53 v76.2,66.24
  Bottom 0.203: v61.37,79.05 67.67,79.05 68.07,79.45 70.92,79.45 v74.37,76 75.18,75.18 75.18,67.26 v76.2,66.24 | v78.23,27.43 78.23,27.84 78.03,28.04 78.03,34.54 79.25,35.76 79.25,35.97 81.08,37.8 v81.48,37.8
SDA_5.0V  (via drill 0.41)
  Top 0.203: 58.12,73.76 58.12,71.53 59.13,70.51 SERIAL.3 | 58.12,73.76 58.12,76.81 Q1.3 | v67.06,41.86 67.46,42.27 67.46,42.88 U$23.23 | 68.89,74.98 69.9,76 R2.1 | 68.89,74.98 v67.67,73.76 58.12,73.76 | 68.89,74.98 73.56,74.98 78.03,70.51 78.84,70.51 SERIAL2.3
  Bottom 0.203: v67.06,41.86 67.06,44.91 67.67,45.52 v67.67,73.76
TXD0_3.3V  (via drill 0.41)
  Top 0.203: v71.53,27.03 67.06,31.5 65.63,31.5 U3.9 | v74.17,19.51 v74.17,24.38
  Bottom 0.203: v74.17,24.38 v71.53,27.03 | v74.17,19.51 74.17,10.77 75.39,9.55 B1.P1-8
TXD0_5.0V  (via drill 0.41)
  Top 0.203: v69.49,35.76 69.7,35.56 69.7,34.34 69.49,34.14 65.43,34.14 64.21,32.92 64.21,31.7 U3.10
  Bottom 0.203: v69.49,35.76 69.49,42.67 74.78,47.95 74.78,49.38 UART1.3
VIN
  Top 0.508: IC1.3 23.77,9.55 20.73,9.55 20.32,9.14 D1.C 20.73,9.75 17.68,12.8 17.68,13.01 | 17.68,13.01 18.69,13.01 18.9,12.8 PC1.+ | 17.68,13.01 15.04,13.01 C2.1

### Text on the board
_tsilk: PCB-RPIBO1 | v11-13 | 5V | GND | 5V
_bsilk: GITHUB: SKAARHOJ-Open-Engineering

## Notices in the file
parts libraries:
SparkFun: Licensing: CC v3.0 Share-Alike You are welcome to use this library for commercial purposes.
